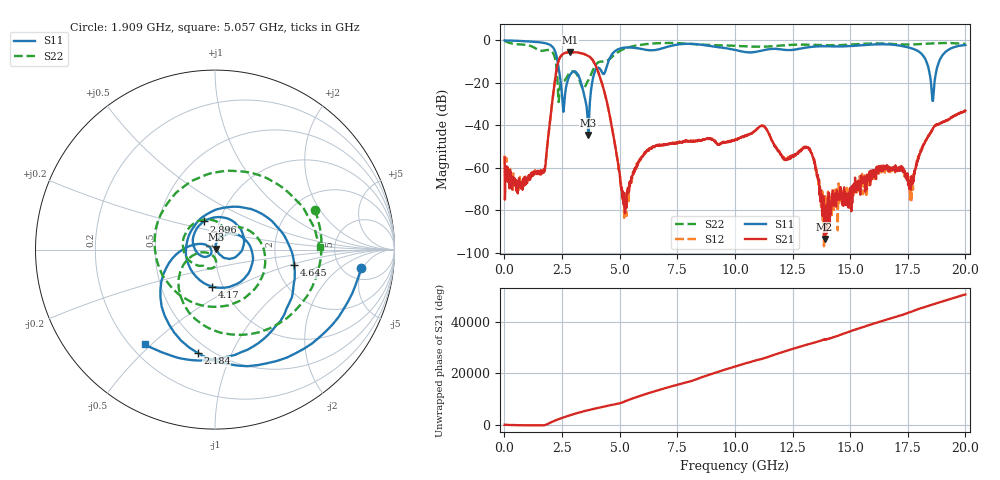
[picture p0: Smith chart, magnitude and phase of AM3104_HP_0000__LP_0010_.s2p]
!Created with skrf (http://scikit-rf.org).
# Hz S RI R 50.0
!freq ReS11 ImS11 ReS21 ImS21 ReS12 ImS12 ReS22 ImS22
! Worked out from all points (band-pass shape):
!   1601 points, 10 MHz to 20 GHz, reference 50 ohm
!   highest |S21| = -5.48 dB at 2.846 GHz (marker M1); lowest = -93.6 dB at 13.89 GHz (marker M2)
!   |S21| within 3 dB of the highest: 2.39 GHz to 3.772 GHz (1.382 GHz wide, 44.9 % of centre)
!   lowest |S11| = -44.5 dB at 3.646 GHz (marker M3), VSWR 1.01, Z = 50.5 + j0.35 ohm
!   |S11| at or under -10 dB: 2.31 GHz to 4.508 GHz (2.198 GHz wide, 64.5 % of centre); 18.31 GHz to 18.86 GHz (547.8 MHz wide, 2.95 % of centre)
!   |S22| runs from -29.0 to -0.2 dB; largest |S21 - S12| = 0.0034
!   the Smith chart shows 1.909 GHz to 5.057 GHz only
!   S11 on the Smith chart (normalised r, x): 1.909 GHz: 7.19, -4.56; 2.184 GHz: 0.43, -0.75; 2.896 GHz: 0.84, +0.27; 4.17 GHz: 0.89, -0.38; 4.645 GHz: 2.50, -0.55; 5.057 GHz: 0.26, -0.48
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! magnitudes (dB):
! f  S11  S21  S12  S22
! 10 MHz  0.0  -55.3  -54.2  -0.2
! 1.647 GHz  -1.1  -61.6  -62.1  -4.9
! 1.909 GHz  -1.7  -44.6  -44.9  -4.5
! 2.184 GHz  -4.7  -19.6  -19.6  -7.9
! 2.546 GHz  -33.0  -6.4  -6.4  -19.2
! 2.846 GHz  -16.3  -5.5  -5.5  -15.1
! 2.896 GHz  -15.5  -5.5  -5.5  -14.7
! 3.346 GHz  -20.7  -6.1  -6.1  -21.6
! 3.646 GHz  -44.5  -7.4  -7.4  -18.7
! 4.17 GHz  -13.7  -18.0  -18.0  -10.0
! 4.645 GHz  -6.9  -39.6  -39.6  -8.0
! 5.057 GHz  -3.6  -69.0  -67.0  -4.7
! 5.27 GHz  -3.3  -74.7  -79.9  -3.6
! 6.682 GHz  -4.2  -49.4  -49.6  -1.3
! 10.01 GHz  -4.4  -46.8  -47.0  -2.5
! 13.34 GHz  -3.0  -53.4  -53.2  -2.1
! 13.89 GHz  -2.7  -93.6  -78.9  -2.2
! 16.68 GHz  -1.8  -61.4  -59.6  -1.5
! 17.66 GHz  -3.7  -66.5  -67.8  -1.9
! 18.59 GHz  -28.5  -41.6  -41.5  -1.4
! 19.03 GHz  -6.7  -38.3  -38.5  -1.2
! 20 GHz  -2.2  -33.1  -33.2  -1.6
